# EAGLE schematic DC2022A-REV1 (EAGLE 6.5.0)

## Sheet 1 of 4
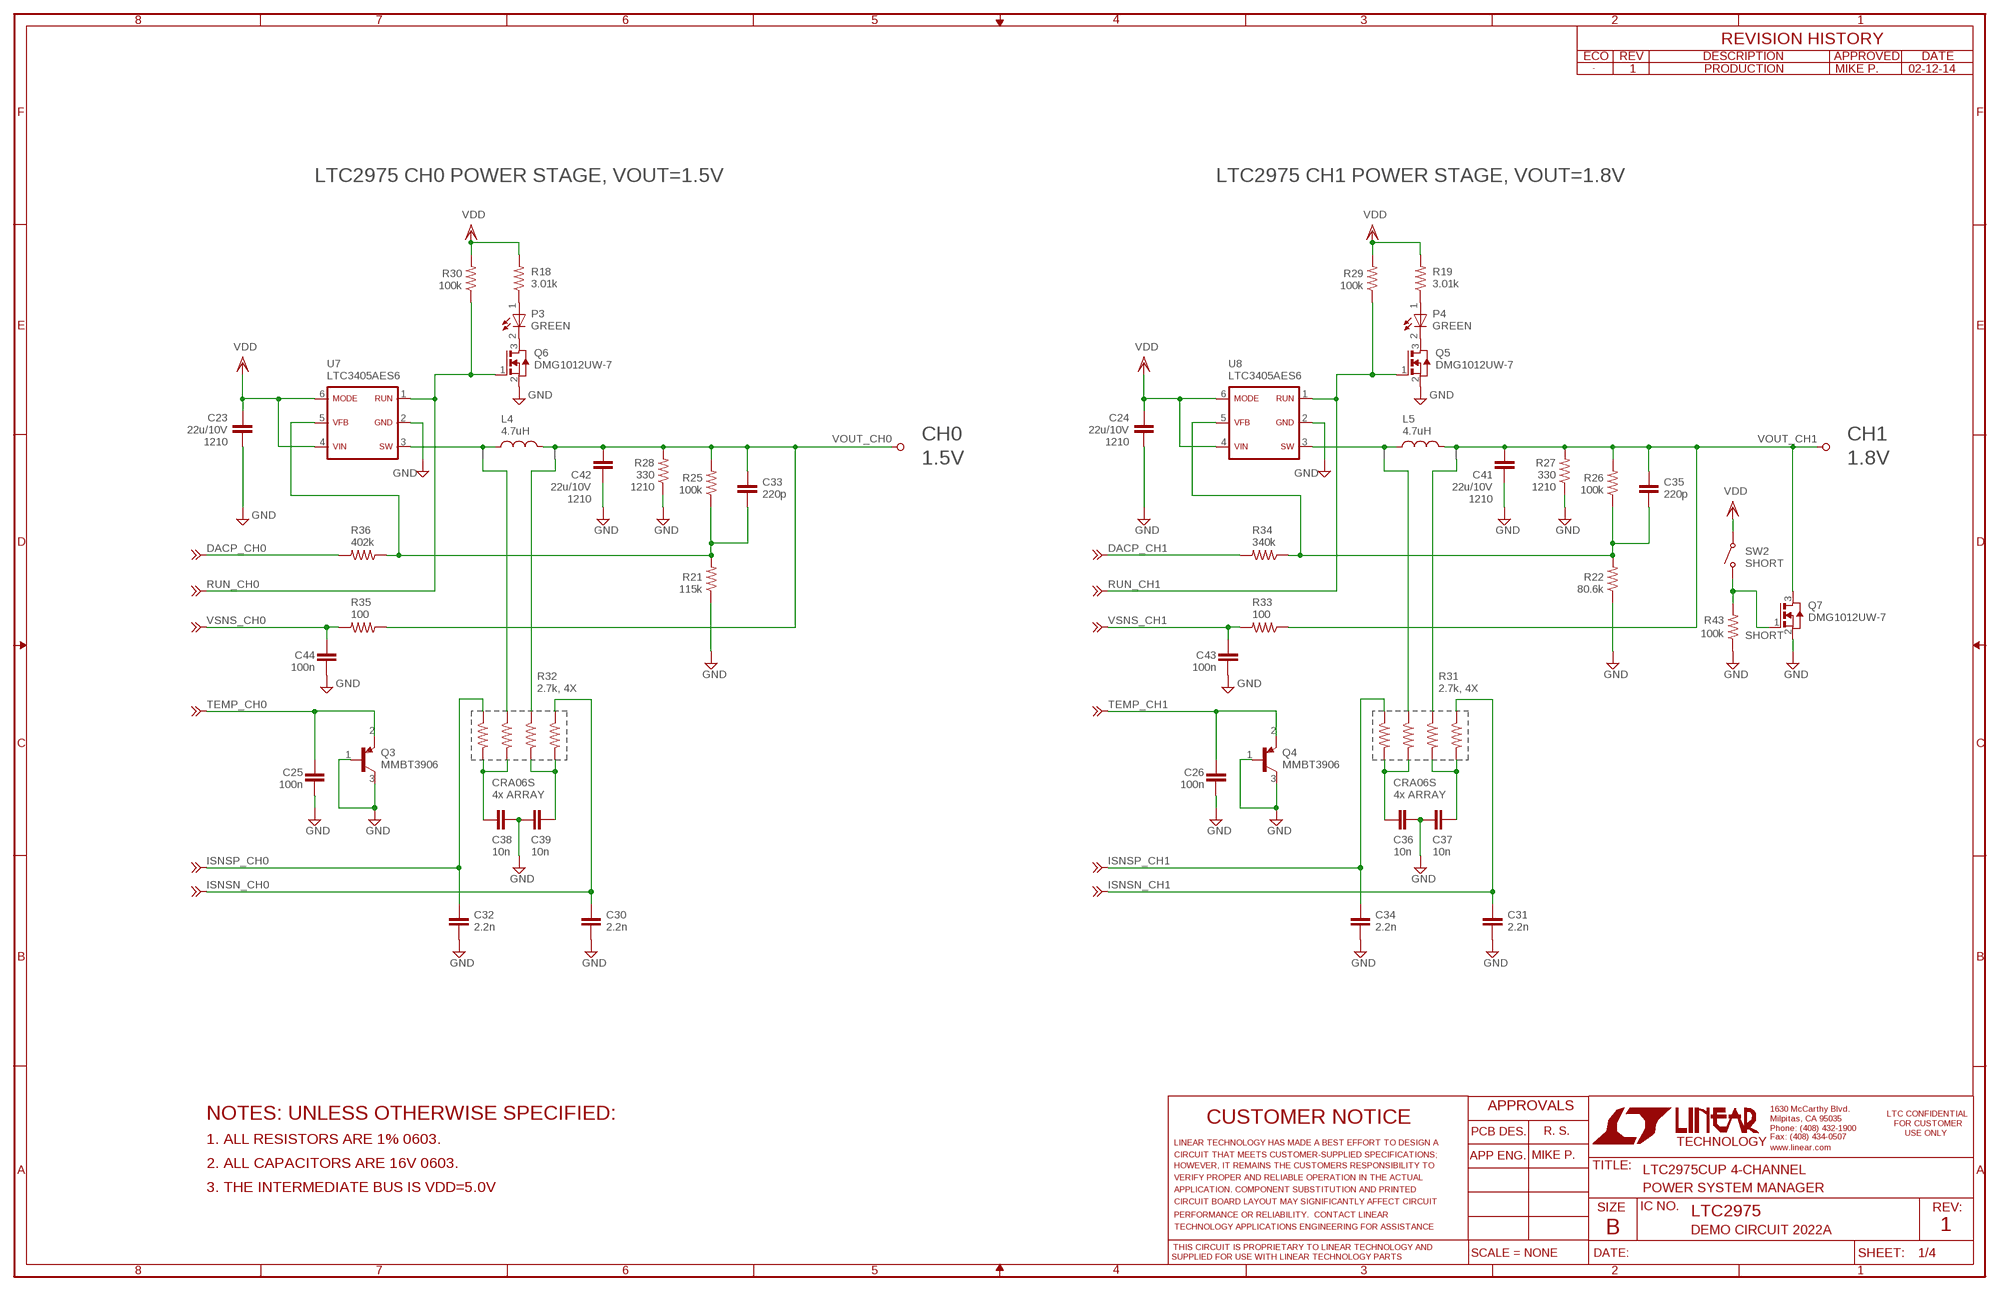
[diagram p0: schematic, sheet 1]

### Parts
C23  22u/10V  CC1210_BOX  [C1210_BOX]
C24  22u/10V  CC1210_BOX  [C1210_BOX]
C25  100n  CC0603_BOX  [C0603_BOX]
C26  100n  CC0603_BOX  [C0603_BOX]
C30  2.2n  CC0603_BOX  [C0603_BOX]
C31  2.2n  CC0603_BOX  [C0603_BOX]
C32  2.2n  CC0603_BOX  [C0603_BOX]
C33  220p  CC0603_BOX  [C0603_BOX]
C34  2.2n  CC0603_BOX  [C0603_BOX]
C35  220p  CC0603_BOX  [C0603_BOX]
C36  10n  CC0603_BOX  [C0603_BOX]
C37  10n  CC0603_BOX  [C0603_BOX]
C38  10n  CC0603_BOX  [C0603_BOX]
C39  10n  CC0603_BOX  [C0603_BOX]
C41  22u/10V  CC1210_BOX  [C1210_BOX]
C42  22u/10V  CC1210_BOX  [C1210_BOX]
C43  100n  CC0603_BOX  [C0603_BOX]
C44  100n  CC0603_BOX  [C0603_BOX]
L4  4.7uH  LL1210  [L1210]
L5  4.7uH  LL1210  [L1210]
NB7  NODE_BREAKER  [NODE_BREAKER]
NB8  NODE_BREAKER  [NODE_BREAKER]
NB9  NODE_BREAKER  [NODE_BREAKER]
NB10  NODE_BREAKER  [NODE_BREAKER]
P3  GREEN  LED-0603  [CHIPLED_0603]
P4  GREEN  LED-0603  [CHIPLED_0603]
Q3  MMBT3906  PNP-SC70  [SC70-3]
Q4  MMBT3906  PNP-SC70  [SC70-3]
Q5  DMG1012UW-7  SI1304  [SC70-3]
Q6  DMG1012UW-7  SI1304  [SC70-3]
Q7  DMG1012UW-7  SI1304  [SC70-3]
R18  3.01k  RR0603_BOX  [R0603_BOX]
R19  3.01k  RR0603_BOX  [R0603_BOX]
R21  115k  RR0603_BOX  [R0603_BOX]
R22  80.6k  RR0603_BOX  [R0603_BOX]
R25  100k  RR0603_BOX  [R0603_BOX]
R26  100k  RR0603_BOX  [R0603_BOX]
R27  330  RR1210_BOX  [R1210_BOX]
R28  330  RR1210_BOX  [R1210_BOX]
R29  100k  RR0603_BOX  [R0603_BOX]
R30  100k  RR0603_BOX  [R0603_BOX]
R31  2.7k, 4X  R_ARRAY_4X_CRA06S  [R_VISHAY_CRA06S]
R32  2.7k, 4X  R_ARRAY_4X_CRA06S  [R_VISHAY_CRA06S]
R33  100  RR0603_BOX  [R0603_BOX]
R34  340k  RR0603_BOX  [R0603_BOX]
R35  100  RR0603_BOX  [R0603_BOX]
R36  402k  RR0603_BOX  [R0603_BOX]
R43  100k  RR0603_BOX  [R0603_BOX]
SW2  PTS635SK25SMTR LFS  SWITCH_PTS635  [SWITCH_PTS635]
TP15  TESPOINT_SMD  TESPOINT_SMDVIA  [VIA]
TP16  TESPOINT_SMD  TESPOINT_SMDVIA  [VIA]
TP17  TESPOINT_SMD  TESPOINT_SMDVIA  [VIA]
TP18  TESPOINT_SMD  TESPOINT_SMDVIA  [VIA]
TP21  TESTPOINT_BIG  [TP1]
TP22  TESTPOINT_BIG  [TP1]
TP23  TESPOINT_SMD  TESPOINT_SMDVIA  [VIA]
TP24  TESPOINT_SMD  TESPOINT_SMDVIA  [VIA]
TP25  TESPOINT_SMD  TESPOINT_SMDVIA  [VIA]
TP26  TESPOINT_SMD  TESPOINT_SMDVIA  [VIA]
TP27  TESPOINT_SMD  TESPOINT_SMDVIA  [VIA]
TP28  TESPOINT_SMD  TESPOINT_SMDVIA  [VIA]
TP29  TESPOINT_SMD  TESPOINT_SMDVIA  [VIA]
TP30  TESPOINT_SMD  TESPOINT_SMDVIA  [VIA]
U7  LTC3405AES6  LTC3405ES6  [SOT-23-6]
U8  LTC3405AES6  LTC3405ES6  [SOT-23-6]

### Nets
DACP_CH0: R36.2 TP28.1 ; also sheet 3
DACP_CH1: R34.2 TP24.1 ; also sheet 3
GND: C23.2 C24.2 C25.2 C26.2 C30.2 C31.2 C32.2 C34.2 C36.1 C37.2 C38.1 C39.2 C41.2 C42.2 C43.1 C44.1 Q3.1(B) Q3.3(C) Q4.1(B) Q4.3(C) Q5.2(S) Q6.2(S) Q7.2(S) R21.1 R22.1 R27.1 R28.1 R43.1 U7.2 U8.2 ; also sheet 2,3,4
ISNSN_CH0: C30.1 R32.R4_1 TP30.1 ; also sheet 3
ISNSN_CH1: C31.1 R31.R4_1 TP26.1 ; also sheet 3
ISNSP_CH0: C32.1 R32.R1_1 TP29.1 ; also sheet 3
ISNSP_CH1: C34.1 R31.R1_1 TP25.1 ; also sheet 3
N$9: P4.P(A) R19.1
N$10: P4.N(C) Q5.3(D)
N$11: C37.1 R31.R3_2 R31.R4_2
N$12: C36.2 R31.R1_2 R31.R2_2
N$13: NB10.1 R31.R3_1
N$14: P3.P(A) R18.1
N$15: P3.N(C) Q6.3(D)
N$16: C39.1 R32.R3_2 R32.R4_2
N$17: C38.2 R32.R1_2 R32.R2_2
N$18: NB9.1 R32.R3_1
RUN_CH0: Q6.1(G) R30.1 TP16.1 U7.1 ; also sheet 3
RUN_CH1: Q5.1(G) R29.1 TP18.1 U8.1 ; also sheet 3
SHORT: Q7.1(G) R43.2 SW2.SW1 ; also sheet 4
SW2: NB8.1 R31.R2_1
SW3: L5.1 NB8.2 U8.3
SW4: NB7.1 R32.R2_1
SW5: L4.1 NB7.2 U7.3
TEMP_CH0: C25.1 Q3.2(E) TP15.1 ; also sheet 3
TEMP_CH1: C26.1 Q4.2(E) TP17.1 ; also sheet 3
VDD: C23.1 C24.1 R18.2 R19.2 R29.2 R30.2 SW2.SW2 U7.4 U7.6 U8.4 U8.6 ; also sheet 2,3
VFB: C35.2 R22.2 R26.1 R34.1 U8.5
VFB1: C33.2 R21.2 R25.1 R36.1 U7.5
VOUT_CH0: C33.1 C42.1 L4.2 NB9.2 R25.2 R28.2 R35.1 TP21.TP
VOUT_CH1: C35.1 C41.1 L5.2 NB10.2 Q7.3(D) R26.2 R27.2 R33.1 TP22.TP
VSNS_CH0: C44.2 R35.2 TP27.1 ; also sheet 3
VSNS_CH1: C43.2 R33.2 TP23.1 ; also sheet 3

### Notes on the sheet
- 1 | PRODUCTION | MIKE P. | 02-12-14
- LTC2975 CH0 POWER STAGE, VOUT=1.5V | LTC2975 CH1 POWER STAGE, VOUT=1.8V
- 1210 | CH0 | 1210 | CH1
- 1.5V | 1.8V
- 1210 | 1210
- 1210 | 1210
- CRA06S | CRA06S
- 4x ARRAY | 4x ARRAY
- NOTES: UNLESS OTHERWISE SPECIFIED:
- R. S.
- 1. ALL RESISTORS ARE 1% 0603.
- MIKE P.
- 2. ALL CAPACITORS ARE 16V 0603.
- LTC2975CUP 4-CHANNEL
- 3. THE INTERMEDIATE BUS IS VDD=5.0V | POWER SYSTEM MANAGER
- LTC2975
- DEMO CIRCUIT 2022A | 1

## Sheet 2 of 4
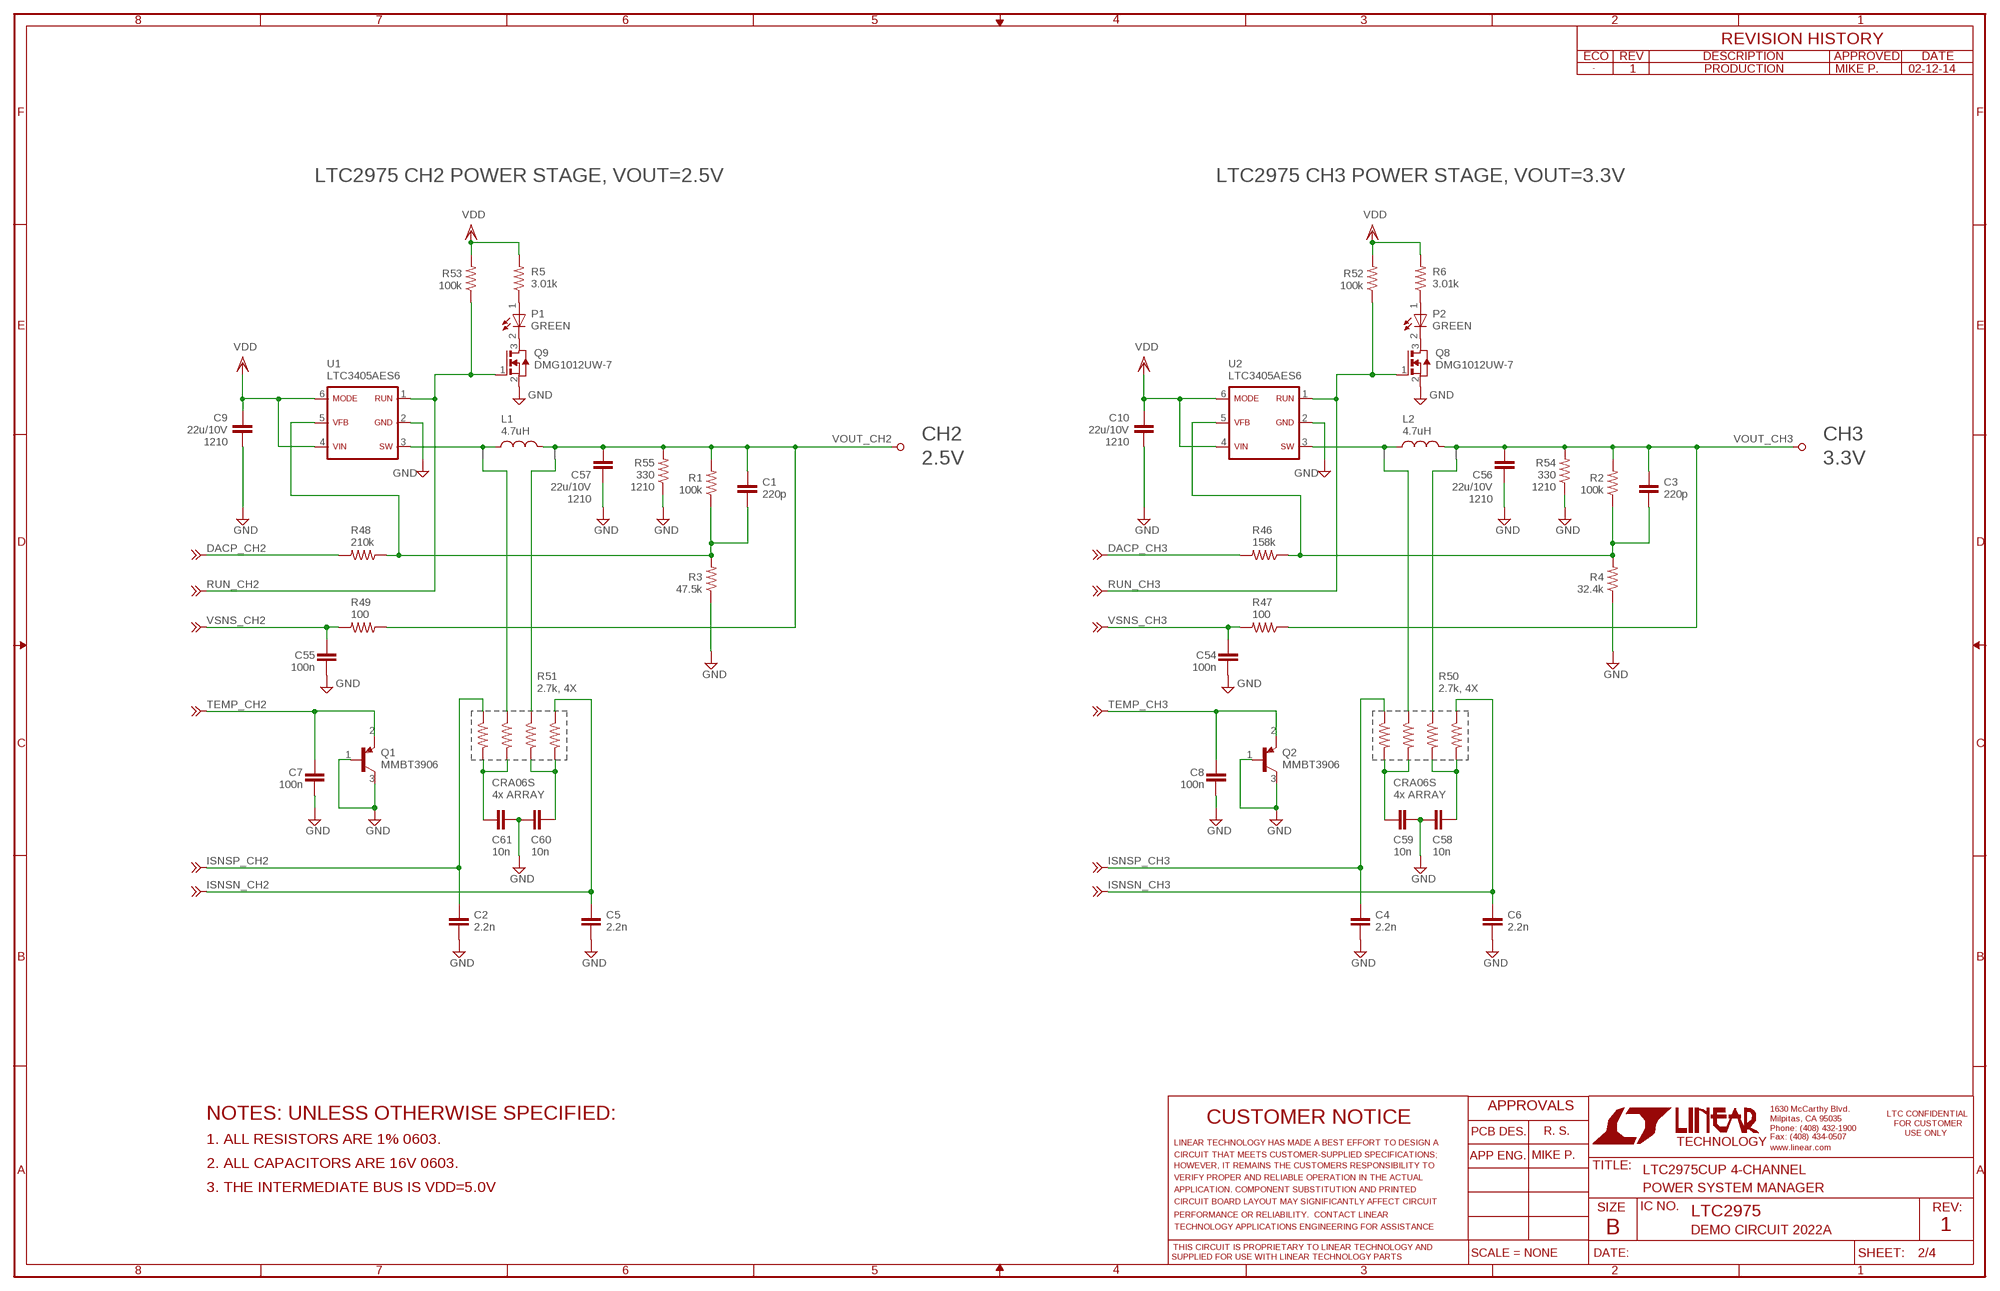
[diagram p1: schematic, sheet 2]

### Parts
C1  220p  CC0603_BOX  [C0603_BOX]
C2  2.2n  CC0603_BOX  [C0603_BOX]
C3  220p  CC0603_BOX  [C0603_BOX]
C4  2.2n  CC0603_BOX  [C0603_BOX]
C5  2.2n  CC0603_BOX  [C0603_BOX]
C6  2.2n  CC0603_BOX  [C0603_BOX]
C7  100n  CC0603_BOX  [C0603_BOX]
C8  100n  CC0603_BOX  [C0603_BOX]
C9  22u/10V  CC1210_BOX  [C1210_BOX]
C10  22u/10V  CC1210_BOX  [C1210_BOX]
C54  100n  CC0603_BOX  [C0603_BOX]
C55  100n  CC0603_BOX  [C0603_BOX]
C56  22u/10V  CC1210_BOX  [C1210_BOX]
C57  22u/10V  CC1210_BOX  [C1210_BOX]
C58  10n  CC0603_BOX  [C0603_BOX]
C59  10n  CC0603_BOX  [C0603_BOX]
C60  10n  CC0603_BOX  [C0603_BOX]
C61  10n  CC0603_BOX  [C0603_BOX]
L1  4.7uH  LL1210  [L1210]
L2  4.7uH  LL1210  [L1210]
NB1  NODE_BREAKER  [NODE_BREAKER]
NB2  NODE_BREAKER  [NODE_BREAKER]
NB3  NODE_BREAKER  [NODE_BREAKER]
NB4  NODE_BREAKER  [NODE_BREAKER]
P1  GREEN  LED-0603  [CHIPLED_0603]
P2  GREEN  LED-0603  [CHIPLED_0603]
Q1  MMBT3906  PNP-SC70  [SC70-3]
Q2  MMBT3906  PNP-SC70  [SC70-3]
Q8  DMG1012UW-7  SI1304  [SC70-3]
Q9  DMG1012UW-7  SI1304  [SC70-3]
R1  100k  RR0603_BOX  [R0603_BOX]
R2  100k  RR0603_BOX  [R0603_BOX]
R3  47.5k  RR0603_BOX  [R0603_BOX]
R4  32.4k  RR0603_BOX  [R0603_BOX]
R5  3.01k  RR0603_BOX  [R0603_BOX]
R6  3.01k  RR0603_BOX  [R0603_BOX]
R46  158k  RR0603_BOX  [R0603_BOX]
R47  100  RR0603_BOX  [R0603_BOX]
R48  210k  RR0603_BOX  [R0603_BOX]
R49  100  RR0603_BOX  [R0603_BOX]
R50  2.7k, 4X  R_ARRAY_4X_CRA06S  [R_VISHAY_CRA06S]
R51  2.7k, 4X  R_ARRAY_4X_CRA06S  [R_VISHAY_CRA06S]
R52  100k  RR0603_BOX  [R0603_BOX]
R53  100k  RR0603_BOX  [R0603_BOX]
R54  330  RR1210_BOX  [R1210_BOX]
R55  330  RR1210_BOX  [R1210_BOX]
TP3  TESTPOINT_BIG  [TP1]
TP4  TESTPOINT_BIG  [TP1]
TP8  TESPOINT_SMD  TESPOINT_SMDVIA  [VIA]
TP9  TESPOINT_SMD  TESPOINT_SMDVIA  [VIA]
TP10  TESPOINT_SMD  TESPOINT_SMDVIA  [VIA]
TP11  TESPOINT_SMD  TESPOINT_SMDVIA  [VIA]
TP31  TESPOINT_SMD  TESPOINT_SMDVIA  [VIA]
TP32  TESPOINT_SMD  TESPOINT_SMDVIA  [VIA]
TP33  TESPOINT_SMD  TESPOINT_SMDVIA  [VIA]
TP34  TESPOINT_SMD  TESPOINT_SMDVIA  [VIA]
TP35  TESPOINT_SMD  TESPOINT_SMDVIA  [VIA]
TP36  TESPOINT_SMD  TESPOINT_SMDVIA  [VIA]
TP37  TESPOINT_SMD  TESPOINT_SMDVIA  [VIA]
TP38  TESPOINT_SMD  TESPOINT_SMDVIA  [VIA]
U1  LTC3405AES6  LTC3405ES6  [SOT-23-6]
U2  LTC3405AES6  LTC3405ES6  [SOT-23-6]

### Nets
DACP_CH2: R48.2 TP37.1 ; also sheet 3
DACP_CH3: R46.2 TP33.1 ; also sheet 3
GND: C2.2 C4.2 C5.2 C6.2 C7.2 C8.2 C9.2 C10.2 C54.1 C55.1 C56.2 C57.2 C58.2 C59.1 C60.2 C61.1 Q1.1(B) Q1.3(C) Q2.1(B) Q2.3(C) Q8.2(S) Q9.2(S) R3.1 R4.1 R54.1 R55.1 U1.2 U2.2 ; also sheet 1,3,4
ISNSN_CH2: C5.1 R51.R4_1 TP35.1 ; also sheet 3
ISNSN_CH3: C6.1 R50.R4_1 TP31.1 ; also sheet 3
ISNSP_CH2: C2.1 R51.R1_1 TP36.1 ; also sheet 3
ISNSP_CH3: C4.1 R50.R1_1 TP32.1 ; also sheet 3
N$19: P1.P(A) R5.1
N$20: P1.N(C) Q9.3(D)
N$21: C60.1 R51.R3_2 R51.R4_2
N$22: C61.2 R51.R1_2 R51.R2_2
N$23: NB1.1 R51.R3_1
N$24: P2.P(A) R6.1
N$25: P2.N(C) Q8.3(D)
N$26: C58.1 R50.R3_2 R50.R4_2
N$27: C59.2 R50.R1_2 R50.R2_2
N$28: NB2.1 R50.R3_1
RUN_CH2: Q9.1(G) R53.1 TP8.1 U1.1 ; also sheet 3
RUN_CH3: Q8.1(G) R52.1 TP10.1 U2.1 ; also sheet 3
SW7: NB3.1 R51.R2_1
SW8: L1.1 NB3.2 U1.3
SW9: NB4.1 R50.R2_1
SW10: L2.1 NB4.2 U2.3
TEMP_CH2: C7.1 Q1.2(E) TP9.1 ; also sheet 3
TEMP_CH3: C8.1 Q2.2(E) TP11.1 ; also sheet 3
VDD: C9.1 C10.1 R5.2 R6.2 R52.2 R53.2 U1.4 U1.6 U2.4 U2.6 ; also sheet 1,3
VFB2: C1.2 R1.1 R3.2 R48.1 U1.5
VFB3: C3.2 R2.1 R4.2 R46.1 U2.5
VOUT_CH2: C1.1 C57.1 L1.2 NB1.2 R1.2 R49.1 R55.2 TP3.TP
VOUT_CH3: C3.1 C56.1 L2.2 NB2.2 R2.2 R47.1 R54.2 TP4.TP
VSNS_CH2: C55.2 R49.2 TP38.1 ; also sheet 3
VSNS_CH3: C54.2 R47.2 TP34.1 ; also sheet 3

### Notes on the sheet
- 1 | PRODUCTION | MIKE P. | 02-12-14
- LTC2975 CH2 POWER STAGE, VOUT=2.5V | LTC2975 CH3 POWER STAGE, VOUT=3.3V
- 1210 | CH2 | 1210 | CH3
- 2.5V | 3.3V
- 1210 | 1210
- 1210 | 1210
- CRA06S | CRA06S
- 4x ARRAY | 4x ARRAY
- NOTES: UNLESS OTHERWISE SPECIFIED:
- R. S.
- 1. ALL RESISTORS ARE 1% 0603.
- MIKE P.
- 2. ALL CAPACITORS ARE 16V 0603.
- LTC2975CUP 4-CHANNEL
- 3. THE INTERMEDIATE BUS IS VDD=5.0V | POWER SYSTEM MANAGER
- LTC2975
- DEMO CIRCUIT 2022A | 1

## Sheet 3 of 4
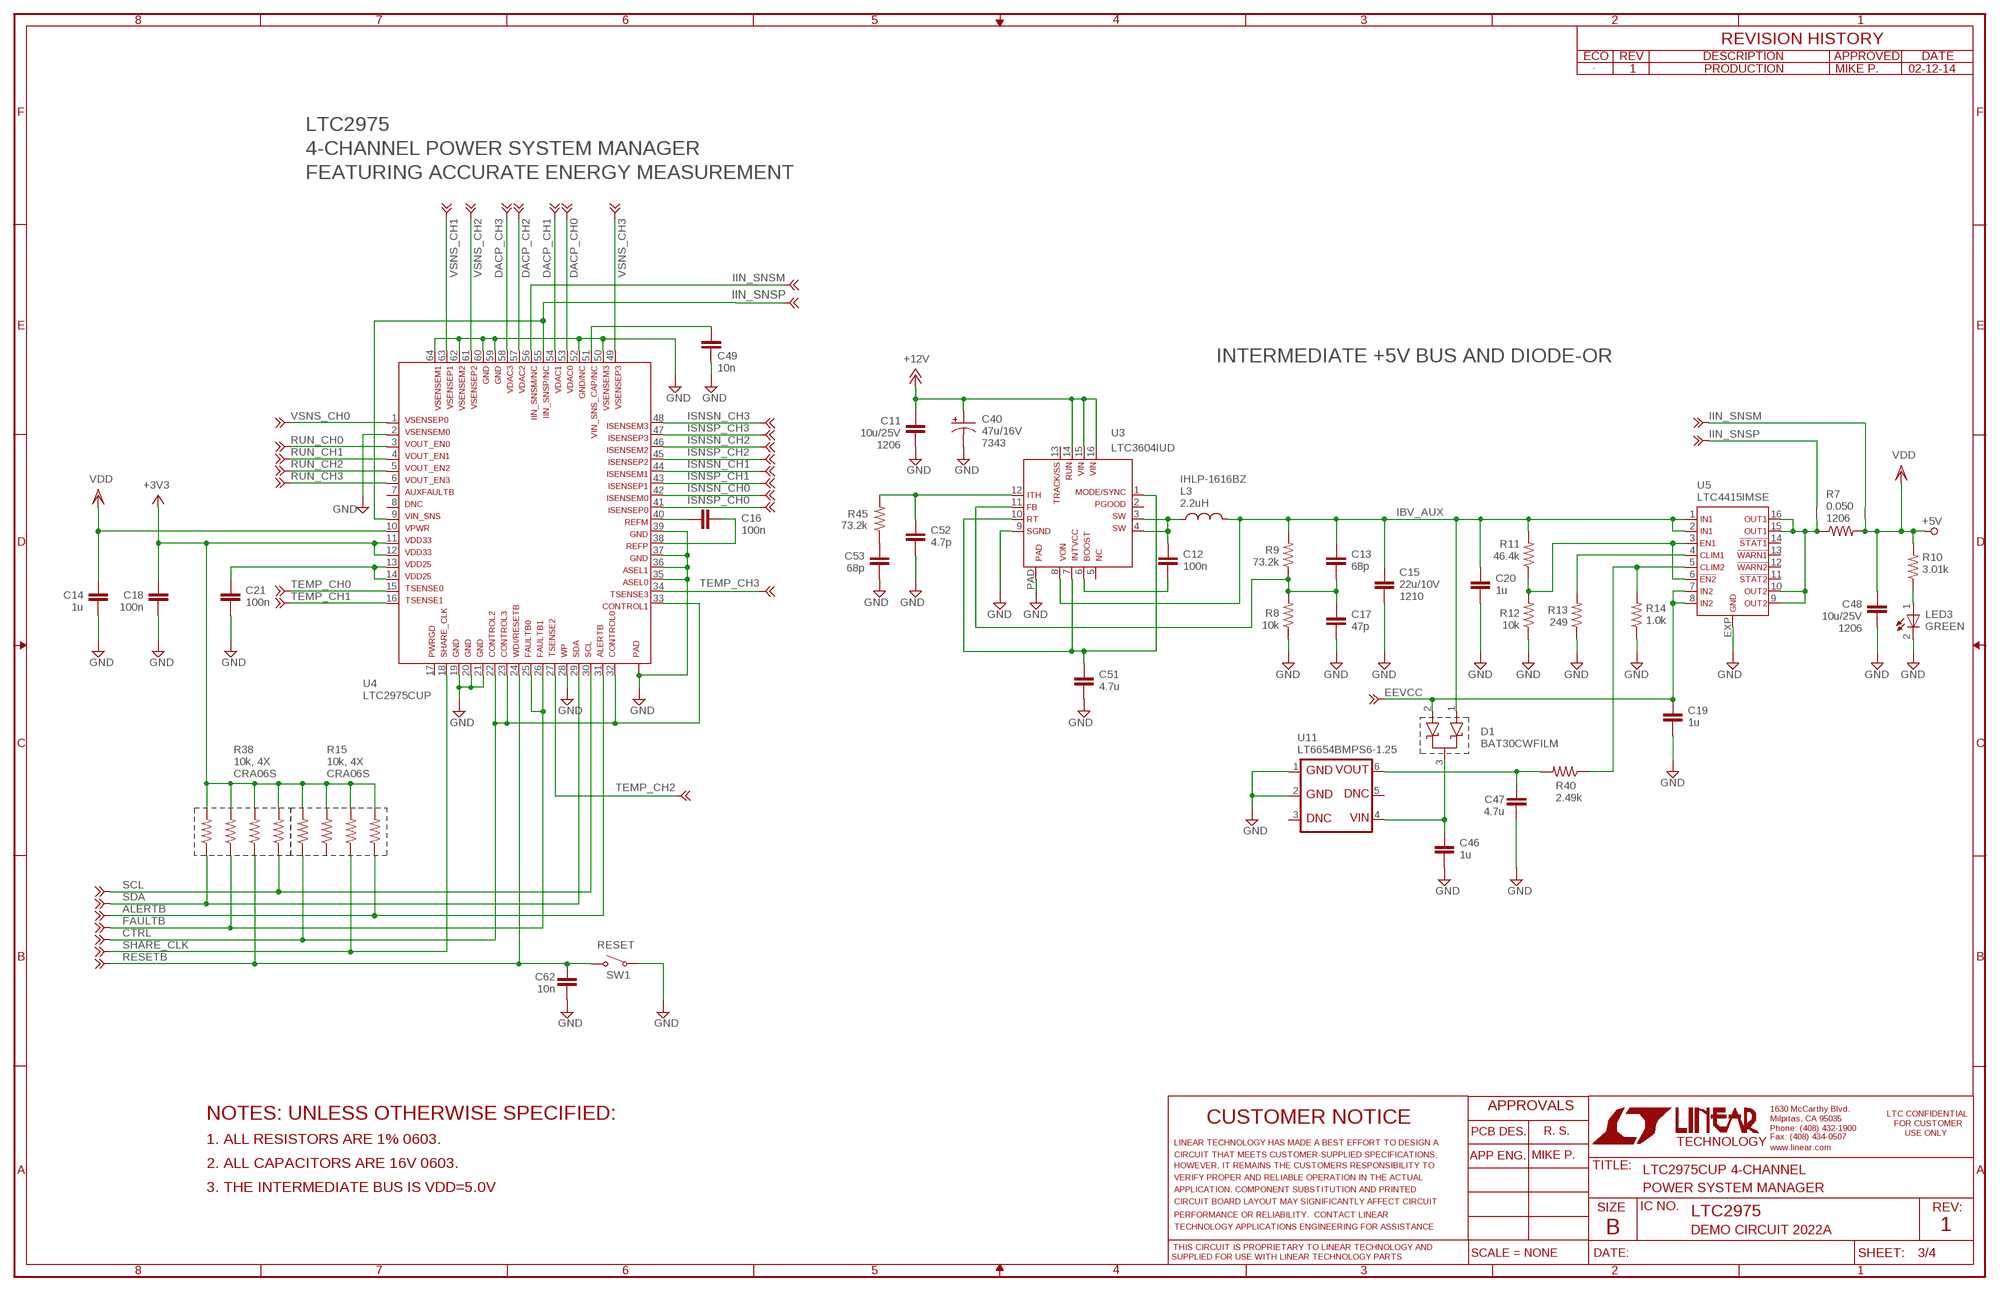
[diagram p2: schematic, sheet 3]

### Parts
C11  10u/25V  CC1206_BOX  [C1206_BOX]
C12  100n  CC0603_BOX  [C0603_BOX]
C13  68p  CC0603_BOX  [C0603_BOX]
C14  1u  CC0603_BOX  [C0603_BOX]
C15  22u/10V  CC1210_BOX  [C1210_BOX]
C16  100n  CC0603_BOX  [C0603_BOX]
C17  47p  CC0603_BOX  [C0603_BOX]
C18  100n  CC0603_BOX  [C0603_BOX]
C19  1u  CC0603_BOX  [C0603_BOX]
C20  1u  CC0603_BOX  [C0603_BOX]
C21  100n  CC0603_BOX  [C0603_BOX]
C40  47u/16V  CPOL  [C7343]
C46  1u  CC0603_BOX  [C0603_BOX]
C47  4.7u  CC0603_BOX  [C0603_BOX]
C48  10u/25V  CC1206_BOX  [C1206_BOX]
C49  10n  CC0603_BOX  [C0603_BOX]
C51  4.7u  CC0603_BOX  [C0603_BOX]
C52  4.7p  CC0603_BOX  [C0603_BOX]
C53  68p  CC0603_BOX  [C0603_BOX]
C62  10n  CC0603_BOX  [C0603_BOX]
D1  BAT30CWFILM  [SC70-3]
L3  2.2uH  LVISHAY-IHLP1616AB  [IHLP_1616AB]
LED3  GREEN  LED-0603  [CHIPLED_0603]
NB5  NODE_BREAKER  [NODE_BREAKER]
NB6  NODE_BREAKER  [NODE_BREAKER]
R7  0.050  RR1206_BOX  [R1206_BOX]
R8  10k  RR0603_BOX  [R0603_BOX]
R9  73.2k  RR0603_BOX  [R0603_BOX]
R10  3.01k  RR0603_BOX  [R0603_BOX]
R11  46.4k  RR0603_BOX  [R0603_BOX]
R12  10k  RR0603_BOX  [R0603_BOX]
R13  249  RR0603_BOX  [R0603_BOX]
R14  1.0k  RR0603_BOX  [R0603_BOX]
R15  10k, 4X  R_ARRAY_4X_CRA06S  [R_VISHAY_CRA06S]
R38  10k, 4X  R_ARRAY_4X_CRA06S  [R_VISHAY_CRA06S]
R40  2.49k  RR0603_BOX  [R0603_BOX]
R45  73.2k  RR0603_BOX  [R0603_BOX]
SW1  PTS635SL25SMTR LFS  SWITCH_PTS635  [SWITCH_PTS635]
TP14  TESTPOINT_BIG  [TP1]
U3  LTC3604IUD  [QFN16_3X3]
U4  LTC2975CUP  LTC2975  [QFN64_9X9]
U5  LTC4415IMSE  [MSOP16_EXP]
U11  LT6654BMPS6-1.25  LTC6654SOT23-6  [SOT-23-6@1]

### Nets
+3V3: C18.2 R15.R1_2 R15.R2_2 R15.R3_2 R15.R4_2 R38.R1_2 R38.R2_2 R38.R3_2 R38.R4_2 U4.11 U4.12 ; also sheet 4
+12V: C11.2 C40.+ U3.14 U3.15 U3.16 ; also sheet 4
ALERTB: R15.R4_1 U4.31 ; also sheet 4
CTRL: R15.R1_1 U4.22 U4.23 U4.32 U4.33 ; also sheet 4
DACP_CH0: U4.53 ; also sheet 1
DACP_CH1: U4.54 ; also sheet 1
DACP_CH2: U4.57 ; also sheet 2
DACP_CH3: U4.58 ; also sheet 2
EEVCC: C19.1 D1.2 U5.7 U5.8 ; also sheet 4
FAULTB: R38.R2_1 U4.25 U4.26 ; also sheet 4
FB_LTC3604: C13.2 C17.1 R8.2 R9.1 U3.11
GND: C11.1 C14.1 C15.2 C17.2 C18.1 C19.2 C20.2 C21.1 C40.- C46.2 C47.1 C48.2 C49.1 C51.2 C52.2 C53.2 C62.1 LED3.N(C) R8.1 R12.1 R13.1 R14.1 SW1.SW2 U3.9 U3.PAD U4.2 U4.19 U4.20 U4.21 U4.28 U4.35 U4.36 U4.37 U4.39 U4.50 U4.52 U4.59 U4.60 U4.62 U4.64 U4.PAD1 U4.PAD2 U4.PAD3 U4.PAD4 U5.EXP U11.1 U11.2 ; also sheet 1,2,4
IBV_AUX: C13.1 C15.1 C20.1 D1.1 L3.2 R9.2 R11.2 U3.8 U5.1 U5.2
IIN_SNSM: NB6.2 U4.56
IIN_SNSP: NB5.2 U4.9 U4.55
INTVCC_LTC3604: C51.1 U3.1 U3.7 U3.10
ISNSN_CH0: U4.42 ; also sheet 1
ISNSN_CH1: U4.44 ; also sheet 1
ISNSN_CH2: U4.46 ; also sheet 2
ISNSN_CH3: U4.48 ; also sheet 2
ISNSP_CH0: U4.41 ; also sheet 1
ISNSP_CH1: U4.43 ; also sheet 1
ISNSP_CH2: U4.45 ; also sheet 2
ISNSP_CH3: U4.47 ; also sheet 2
ITH_LTC3604: C52.1 R45.2 U3.12
N$1: C46.1 D1.3 U11.4
N$48: C16.1 U4.40
N$49: C16.2 U4.38
N$52: C21.2 U4.13 U4.14
N$61: C53.1 R45.1
N$63: LED3.P(A) R10.1
N$64: R14.2 R40.1 U5.5
N$68: R13.2 U5.4
N$69: R11.1 R12.2 U5.3 U5.6
N$70: C12.2 U3.6
RESETB: C62.2 R38.R3_1 SW1.SW1 U4.24 ; also sheet 4
RUN_CH0: U4.3 ; also sheet 1
RUN_CH1: U4.4 ; also sheet 1
RUN_CH2: U4.5 ; also sheet 2
RUN_CH3: U4.6 ; also sheet 2
SCL: R38.R4_1 U4.30 ; also sheet 4
SDA: R38.R1_1 U4.29 ; also sheet 4
SHARE_CLK: R15.R3_1 U4.18 ; also sheet 4
SW_LTC3604: C12.1 L3.1 U3.3 U3.4
TEMP_CH0: U4.15 ; also sheet 1
TEMP_CH1: U4.16 ; also sheet 1
TEMP_CH2: U4.27 ; also sheet 2
TEMP_CH3: U4.34 ; also sheet 2
VDD: C14.2 C48.1 NB6.1 R7.2 R10.2 TP14.TP U4.10 ; also sheet 1,2
VDD_OR: NB5.1 R7.1 U5.9 U5.10 U5.15 U5.16
VIN_SNS_CAP: C49.2 U4.51
VREF: C47.2 R40.2 U11.6
VSNS_CH0: U4.1 ; also sheet 1
VSNS_CH1: U4.63 ; also sheet 1
VSNS_CH2: U4.61 ; also sheet 2
VSNS_CH3: U4.49 ; also sheet 2
Unconnected: R15.R2_1 U3.2 U3.5 U3.13 U4.7 U4.8 U4.17 U5.11 U5.12 U5.13 U5.14 U11.3 U11.5

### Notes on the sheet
- 1 | PRODUCTION | MIKE P. | 02-12-14
- LTC2975
- 4-CHANNEL POWER SYSTEM MANAGER
- FEATURING ACCURATE ENERGY MEASUREMENT
- INTERMEDIATE +5V BUS AND DIODE-OR
- 1206
- 7343
- IHLP-1616BZ
- 1206 | +5V
- 1210
- 1206
- CRA06S | CRA06S
- RESET
- NOTES: UNLESS OTHERWISE SPECIFIED:
- R. S.
- 1. ALL RESISTORS ARE 1% 0603.
- MIKE P.
- 2. ALL CAPACITORS ARE 16V 0603.
- LTC2975CUP 4-CHANNEL
- 3. THE INTERMEDIATE BUS IS VDD=5.0V | POWER SYSTEM MANAGER
- LTC2975
- DEMO CIRCUIT 2022A | 1

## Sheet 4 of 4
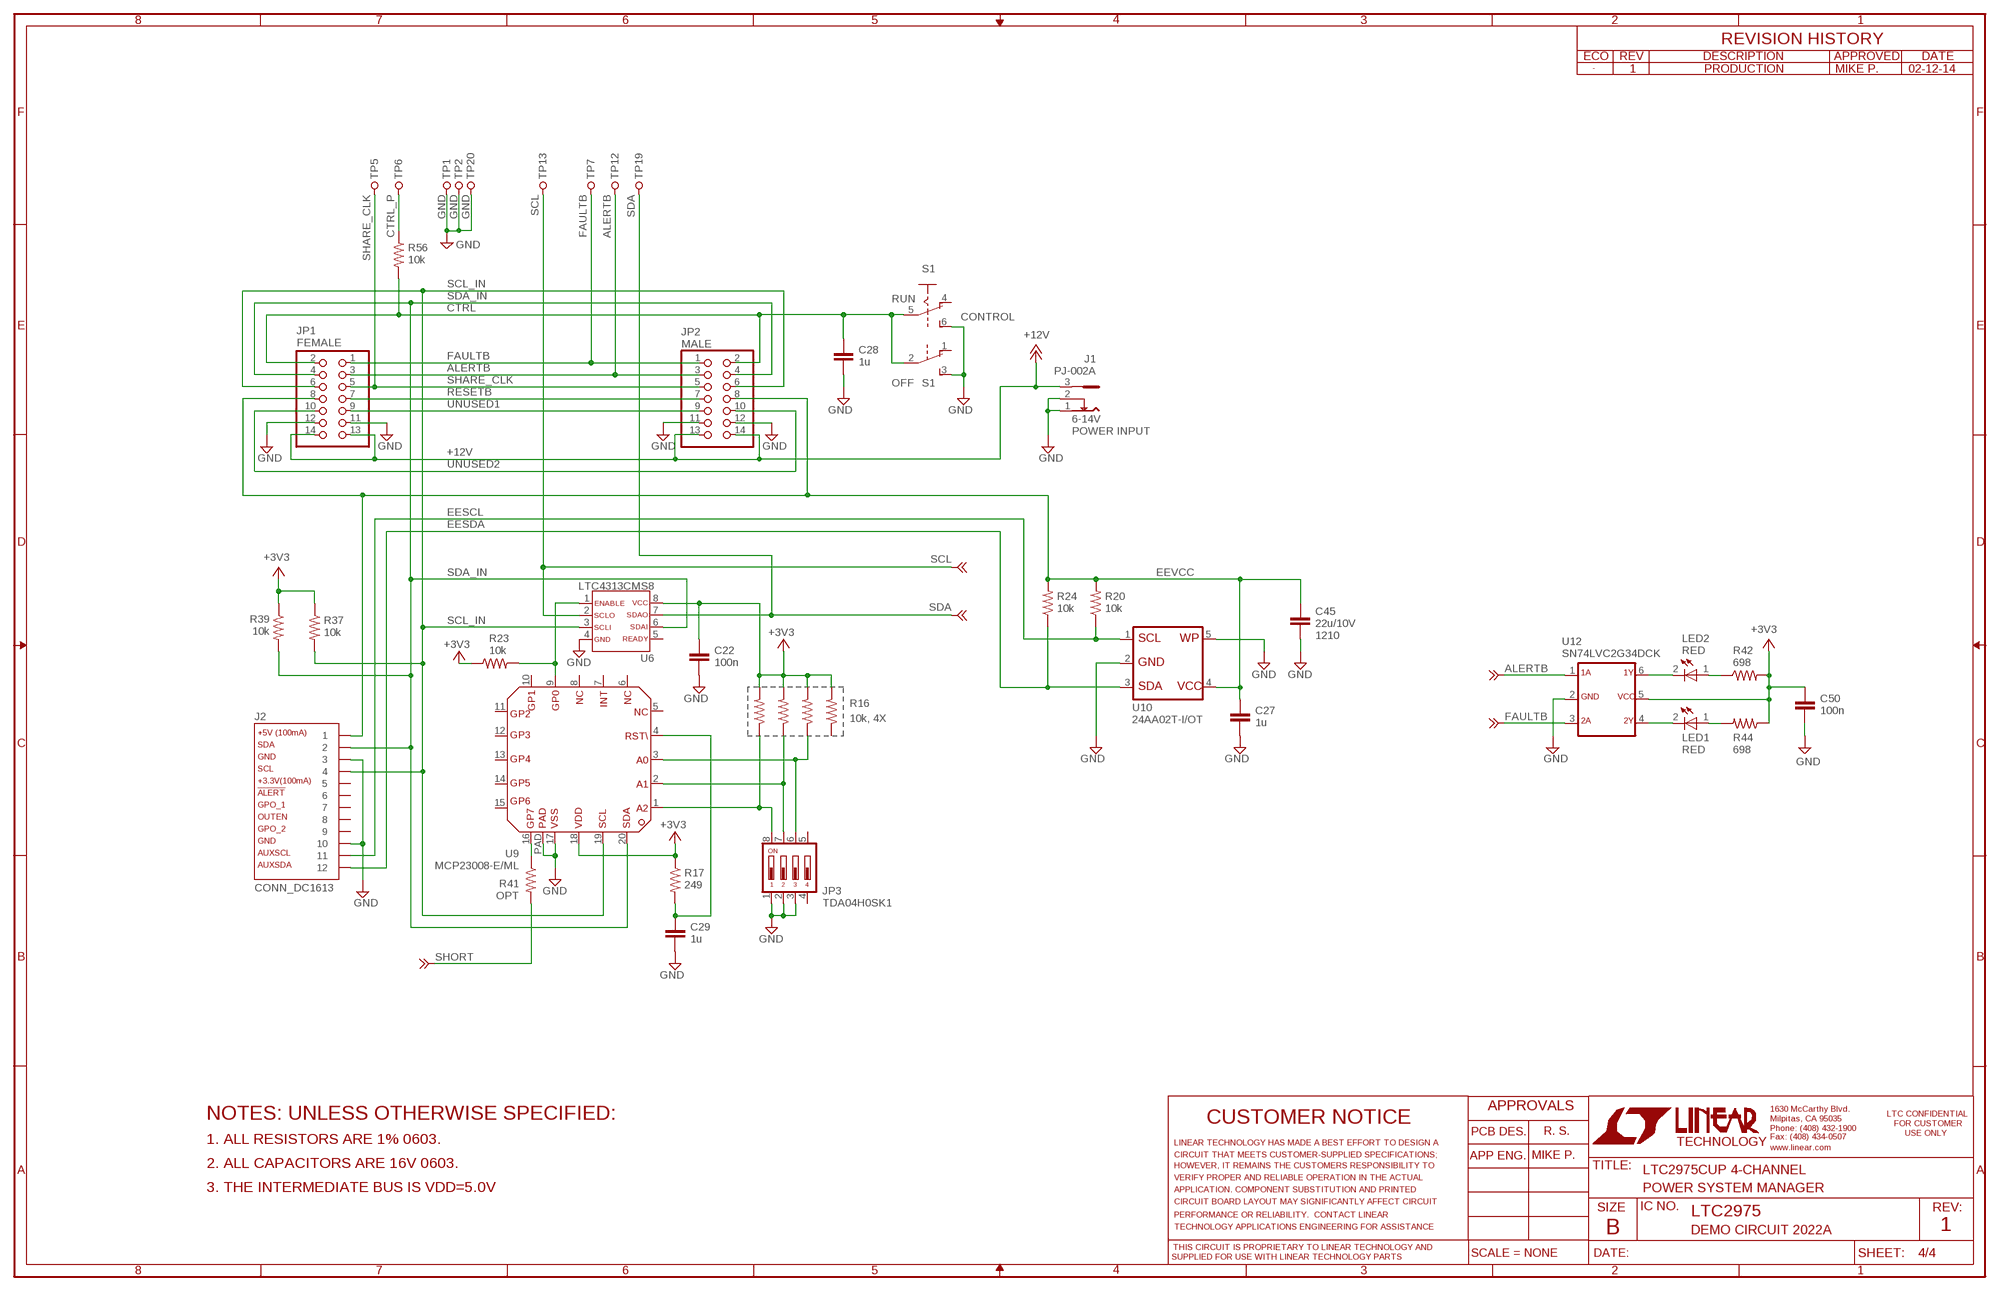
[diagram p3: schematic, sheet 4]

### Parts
C22  100n  CC0603_BOX  [C0603_BOX]
C27  1u  CC0603_BOX  [C0603_BOX]
C28  1u  CC0603_BOX  [C0603_BOX]
C29  1u  CC0603_BOX  [C0603_BOX]
C45  22u/10V  CC1210_BOX  [C1210_BOX]
C50  100n  CC0603_BOX  [C0603_BOX]
J1  PJ-002A  [PJ-002A]
J2  CONN_DC1613  [CONN_DC1613]
JP1  FEMALE  PINHD-2X07_2.00  [2X07M]
JP2  MALE  PINHD-2X07_2.00  [2X07M]
JP3  TDA04H0SK1  [SMT_DIP_4]
LED1  RED  LED-0603  [CHIPLED_0603]
LED2  RED  LED-0603  [CHIPLED_0603]
R16  10k, 4X  R_ARRAY_4X_CRA06S  [R_VISHAY_CRA06S]
R17  249  RR0603_BOX  [R0603_BOX]
R20  10k  RR0603_BOX  [R0603_BOX]
R23  10k  RR0603_BOX  [R0603_BOX]
R24  10k  RR0603_BOX  [R0603_BOX]
R37  10k  RR0603_BOX  [R0603_BOX]
R39  10k  RR0603_BOX  [R0603_BOX]
R41  OPT  RR0603_BOX  [R0603_BOX]
R42  698  RR0603_BOX  [R0603_BOX]
R44  698  RR0603_BOX  [R0603_BOX]
R56  10k  RR0603_BOX  [R0603_BOX]
S1  CONTROL  JS202011CQN  [JS202011CQN]
TP1  TESTPOINT_BIG  [TP1]
TP2  TESTPOINT_BIG  [TP1]
TP5  TESTPOINT_BIG  [TP1]
TP6  TESTPOINT_BIG  [TP1]
TP7  TESTPOINT_BIG  [TP1]
TP12  TESTPOINT_BIG  [TP1]
TP13  TESTPOINT_BIG  [TP1]
TP19  TESTPOINT_BIG  [TP1]
TP20  TESTPOINT_BIG  [TP1]
U6  LTC4313CMS8  [MSOP-8]
U9  MCP23008-E/ML  [QFN20]
U10  24AA02T-I/OT  24AA64  [SOT-23-5]
U12  SN74LVC2G34DCK  [SC70-6]

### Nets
+3V3: C22.1 C50.1 R16.R1_2 R16.R2_2 R16.R3_2 R16.R4_2 R17.1 R23.1 R37.1 R39.1 R42.2 R44.1 U6.8 U9.18 U12.5 ; also sheet 3
+12V: J1.3 JP1.13 JP1.14 JP2.13 JP2.14 ; also sheet 3
A0_MUX: JP3.6 R16.R2_1 U9.3
A1_MUX: JP3.7 R16.R3_1 U9.2
A2_MUX: JP3.8 R16.R4_1 U9.1
ALERTB: JP1.3 JP2.3 TP12.TP U12.1 ; also sheet 3
CTRL: C28.1 JP1.2 JP2.2 R56.2 S1.2(B:P) S1.5(A:P) ; also sheet 3
CTRL_P: R56.1 TP6.TP
EESCL: J2.11 R20.1 U10.1
EESDA: J2.12 R24.1 U10.3
EEVCC: C27.1 C45.1 J2.1 JP1.8 JP2.8 R20.2 R24.2 U10.4 ; also sheet 3
FAULTB: JP1.1 JP2.1 TP7.TP U12.3 ; also sheet 3
GND: C22.2 C27.2 C28.2 C29.2 C45.2 C50.2 J1.1 J1.2 J2.3 J2.10 JP1.11 JP1.12 JP2.11 JP2.12 JP3.1 JP3.2 JP3.3 S1.3(B:S) S1.6(A:S) TP1.TP TP2.TP TP20.TP U6.4 U9.17 U9.PAD U10.2 U10.5 U12.2 ; also sheet 1,2,3
N$3: LED1.P(A) R44.2
N$4: R41.1 U9.16
N$57: LED2.P(A) R42.1
N$58: LED1.N(C) U12.4
N$60: LED2.N(C) U12.6
N$66: C29.1 R17.2 U9.4
N$74: R23.2 U6.1 U9.9
RESETB: JP1.7 JP2.7 ; also sheet 3
SCL: TP13.TP U6.2 ; also sheet 3
SCL_IN: J2.4 JP1.6 JP2.6 R37.2 U6.3 U9.19
SDA: TP19.TP U6.7 ; also sheet 3
SDA_IN: J2.2 JP1.4 JP2.4 R39.2 U6.6 U9.20
SHARE_CLK: JP1.5 JP2.5 TP5.TP ; also sheet 3
SHORT: R41.2 ; also sheet 1
UNUSED1: JP1.9 JP2.9
UNUSED2: JP1.10 JP2.10
Unconnected: J2.5 J2.6 J2.7 J2.8 J2.9 JP3.4 JP3.5 R16.R1_1 S1.1(B:O) S1.4(A:O) U6.5 U9.5 U9.6 U9.7 U9.8 U9.10 U9.11 U9.12 U9.13 U9.14 U9.15

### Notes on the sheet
- 1 | PRODUCTION | MIKE P. | 02-12-14
- RUN
- OFF
- 6-14V
- POWER INPUT
- 1210
- NOTES: UNLESS OTHERWISE SPECIFIED:
- R. S.
- 1. ALL RESISTORS ARE 1% 0603.
- MIKE P.
- 2. ALL CAPACITORS ARE 16V 0603.
- LTC2975CUP 4-CHANNEL
- 3. THE INTERMEDIATE BUS IS VDD=5.0V | POWER SYSTEM MANAGER
- LTC2975
- DEMO CIRCUIT 2022A | 1

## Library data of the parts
C1-C39 C41-C62 = kalin:C: CAPACITOR, European symbol
C40 = kalin:CPOL: Polarized Capacitor
D1 = kalin:BAT30CWFILM: Small signal dual schottky diode (common cathode)
J1 = kalin:PJ-002A: Power Jack from CUI Inc. PJ-002A
J2 = kalin:CONN_DC1613: Connector for LT DC1613 USB Dongle
JP1 JP2 = pinhead_2mm:PINHD-2X07: PIN HEADER
JP3 = kalin:TDA04H0SK1: Ultra-miniature Surface Mount Half-pitch DIP Switch
L1-L5 = kalin:L: Inductor
LED1-LED3 P1-P4 = kalin:LED-0603: SMD LED in R0603
NB1-NB10 = kalin:NODE_BREAKER: NODE_BREAKER
Q1-Q4 = kalin:PNP-SC70: GP PNP transistor in SC70 package
Q5-Q9 = kalin:SI1304: N-Channel 30 V (D-S) MOSFET
R1-R14 R17-R30 R33-R37 R39-R49 R52-R56 = kalin:R: RESISTOR, American symbol
R15 R16 R31 R32 R38 R50 R51 = kalin:R_ARRAY_4X_CRA06S: Thick Film Resistor Array
S1 = kalin:JS202011CQN: SLIDING SWITCH Siemens, distributor Buerklin, 11G766
SW1 SW2 = kalin:SWITCH_PTS635: PTS635SL25 Surface Mount Tactile Switch
TP1-TP7 TP12-TP14 TP19-TP22 = kalin:TESTPOINT_BIG: Large Test Point
TP8-TP11 TP15-TP18 TP23-TP38 = kalin:TESPOINT_SMD: SMALL SMD Test Point
U1 U2 U7 U8 = kalin:LTC3405: 1.5MHz, 300mA Synchronous Step-Down Regulator in ThinSOT
U3 = kalin:LTC3604: 2.5A, 15V Monolithic Synchronous Step-Down Regulator
U4 = kalin:LTC2975: 4-Channel Power System Manager
U5 = kalin:LTC4415: Dual 4A Ideal Diodes with Adjustable Current Limit
U6 = kalin:LTC4313: 2-Wire Bus Buffers with High Noise Margin
U9 = kalin:MCP23008: I2C 8-pin IO Expander
U10 = kalin:24AA64: 64Kbit I2C Serial EEPROM
U11 = kalin:LTC6654: SOT-23 Precision Wide Supply High Output Drive Low Noise Reference
U12 = kalin:SN74LVC2G34: Dual Buffer Gate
